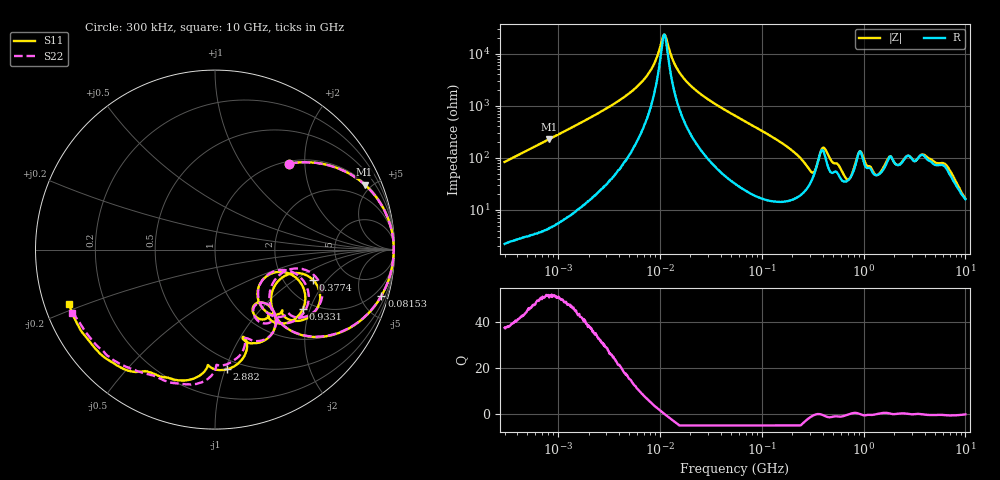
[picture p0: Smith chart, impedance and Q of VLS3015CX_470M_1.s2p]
! S-Parameter Data Generated by TDK Corporation
! Copyright(C) 2019 TDK Corporation.
! All Rights Reserved.
! TDK P/N: VLS3015CX-470M-1 (Inductor)
! Property: L=47uH at 1MHz
! Size(LxWxT): 3x3x1.5mm
! Model Type: s2p (Touchstone File Format Version 1.0)
! Frequency: DC=Yes Start=0.3MHz Stop=10000MHz 802points Log-sweep
! Model Generated on Sep. 23, 2019
! Port Assignments:
!  1 ---@@@--- 2
! Applicable Conditions:
!  Temperature = 25 degC
!  DC Bias Current = 0 A
!  Small Signal Operation
! Terms and conditions regarding TDK Simulation Models
! (1)This simulation model is being provided solely for informational purposes. Please refer to the specifications of the products in terms of detailed characteristics of such products.
! (2)In no event shall TDK Corporation of any of its subsidiaries be liable for any loss or damage arising, directly or indirectly,
!  From any information contained in this simulation model, including, but not limited to loss or damages arising from any inaccuracies, omissions or errors in connection with such information.
! (3)Any and all copyrights on this simulation model are owned by TDK Corporation.
!  Duplication or redistribution of this simulation model without prior written permission from TDK Corporation is prohibited.
! (4)This simulation model is subject to any modification or change without any prior notice.
! (5)Neither TDK Corporation nor any of its subsidiaries shall make any warranty, express or implied,
!  Including but not limited to the correctness, implied warranties of merchantability and fitness for a particular purpose with respect to this simulation models.
! (6)The use of this simulation model shall be deemed to have consented to the terms and conditions hereof.
# Hz S MA R 50
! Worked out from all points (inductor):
!   801 points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, 300 kHz to 10 GHz, reference 50 ohm
!   read as one part in series: L = 44.2 uH near 318.3 kHz
!   highest Q = 51.2 at 820.8 kHz (marker M1), where L = 44.2 uH
!   self-resonance near 11.09 MHz
!   S11 on the Smith chart (normalised r, x): 300 kHz: 1.05, +1.67; 81.53 MHz: 1.03, -7.18; 377.4 MHz: 2.87, -1.44; 933.1 MHz: 1.77, -1.79; 2.882 GHz: 0.42, -1.01; 10 GHz: 0.07, -0.18
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300000  0.6323 49.2  0.7579 -39.2  0.758 -39.2  0.6321 49.2
820758  0.9091 23.5  0.3991 -65.4  0.3992 -65.4  0.9089 23.5
1713600  0.9745 11.6  0.2024 -77.0  0.2024 -77.0  0.9744 11.6
5870124  0.9952 2.4  0.04458 -82.6  0.04456 -82.7  0.9952 2.4
9671944  0.9958 0.2  0.009852 -64.6  0.00986 -64.6  0.9958 0.2
1.125452e7  0.9957 -0.4  0.004372 11.9  0.004376 11.7  0.9957 -0.4
1.421446e7  0.9954 -1.3  0.01679 73.4  0.0168 73.3  0.9954 -1.3
1.80882e7  0.9948 -2.4  0.03322 79.6  0.03323 79.6  0.9949 -2.4
5.477226e7  0.9809 -10.3  0.1521 76.9  0.1521 76.9  0.9808 -10.2
8.153051e7  0.9624 -15.6  0.2302 71.8  0.2302 71.8  0.9623 -15.4
2.102074e8  0.7535 -40.3  0.571 42.6  0.571 42.6  0.7522 -40.2
3.126428e8  0.4071 -39.7  0.6885 8.9  0.6885 8.9  0.3941 -39.6
3.7738e8  0.5722 -17.2  0.438 -3.3  0.4381 -3.3  0.5624 -14.1
4.627802e8  0.5979 -41.7  0.5382 18.8  0.5382 18.8  0.6125 -38.2
6.821612e8  0.3501 -47.4  0.7098 -4.4  0.7098 -4.4  0.3518 -46.9
8.18524e8  0.4009 -18.2  0.5966 -25.1  0.5967 -25.1  0.4023 -16.4
9.330971e8  0.5909 -33.9  0.4109 -14.3  0.4108 -14.3  0.602 -31.2
1.307877e9  0.4165 -58.9  0.6337 -19.9  0.6336 -19.9  0.4164 -58.9
1.767019e9  0.5226 -49.7  0.455 -45.1  0.4548 -45.1  0.5391 -51.0
2.882439e9  0.6705 -84.4  0.3524 -52.6  0.3531 -52.6  0.6397 -83.3
6.41458e9  0.8298 -125.6  0.2264 -72.4  0.2259 -72.5  0.8154 -126.3
1e10  0.8683 -159.6  0.1988 -90.8  0.1991 -90.7  0.8748 -156.0
